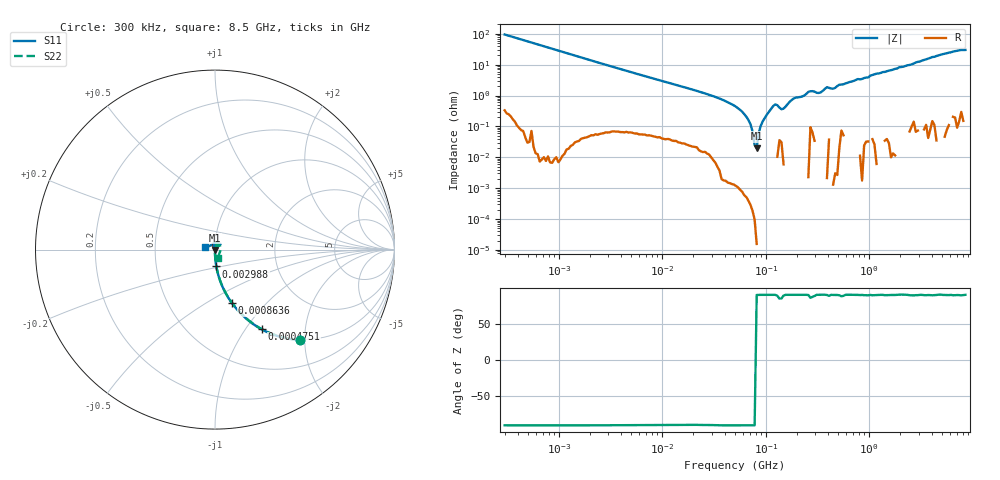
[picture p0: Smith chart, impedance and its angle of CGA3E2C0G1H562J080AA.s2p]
! S-parameter Generated by TDK Corporation
! Copyright(C) 2015 TDK Corporation.
! All Rights Reserved.
! TDK P/N: CGA3E2C0G1H562J080AA (Multilayer Ceramic Chip Capacitors)
! Property: C=5.6nF
! Size(LxWxT): 1.6x0.8x0.8mm, 0.063x0.031x0.031inches
! Model Type: s2p (Touchstone File Format Version 1.0)
! Frequency: DC=Yes Start=0.3MHz Stop=8500MHz 225points Log-sweep
! Note:
! Model Generated on Jun. 23, 2015
! Hash(MD5):
! Port Assignments:
!  1 ---| |--- 2
! Applicable Conditions:
!  Temperature = 25 degC
!  DC Bias Voltage = 0 V
!  Small Signal Operation
! Terms and conditions regarding TDK Simulation Models
! (1)This simulation model is being provided solely for informational purposes. Please refer to the specifications of the products in terms of detailed characteristics of such products.
! (2)In no event shall TDK Corporation of any of its subsidiaries be liable for any loss or damage arising, directly or indirectly,
!  From any information contained in this simulation model, including, but not limited to loss or damages arising from any inaccuracies, omissions or errors in connection with such information.
! (3)Any and all copyrights on this simulation model are owned by TDK Corporation.
!  Duplication or redistribution of this simulation model without prior written permission from TDK Corporation is prohibited.
! (4)This simulation model is subject to any modification or change without any prior notice.
! (5)Neither TDK Corporation nor any of its subsidiaries shall make any warranty, express or implied,
!  Including but not limited to the correctness, implied warranties of merchantability and fitness for a particular purpose with respect to this simulation models.
! (6)The use of this simulation model shall be deemed to have consented to the terms and conditions hereof.
# MHz S MA R 50
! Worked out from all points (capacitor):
!   224 points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, 300 kHz to 8.5 GHz, reference 50 ohm
!   read as one part in series: C = 5.6 nF near 314.1 kHz
!   lowest |Z| = 19.9 mohm at 81.83 MHz (marker M1)
!   series resonance near 80.2 MHz, so ESL is about 700 pH
!   S11 on the Smith chart (normalised r, x): 300 kHz: 0.99, -1.89; 475.1 kHz: 0.99, -1.19; 863.6 kHz: 0.99, -0.66; 2.988 MHz: 1.00, -0.19; 8.5 GHz: 0.90, +0.02
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0.3  0.6902 -46.8  0.7236 43.1  0.7236 43.5  0.6902 -46.7
0.47509  0.515 -59.6  0.8572 30.4  0.8572 30.5  0.515 -59.5
0.8636283  0.3131 -72.4  0.9495 17.8  0.9491 17.8  0.3132 -72.2
1.72111  0.1622 -81.6  0.9859 9.2  0.9824 9.2  0.1626 -81.3
2.988094  0.09404 -85.6  0.9951 5.4  0.9911 5.5  0.09444 -85.2
9.430415  0.0312 -89.2  0.9993 1.7  0.9967 1.9  0.0313 -89.9
51.67171  0.005867 -71.3  1 0.0  1 0.3  0.005867 -108.3
81.82903  0.002481 -46.8  1 -0.2  1 -0.0  0.002481 -133.4
102.9757  0.001212 -39.3  1 -0.4  1 -0.2  0.001212 -141.3
112.8926  0.0003362 -22.9  1 -0.6  1 -0.3  0.0003362 -158.0
178.7805  0.004567 42.9  1 -0.8  1 -0.5  0.004567 135.8
235.5662  0.00314 81.4  1 -1.1  1 -0.9  0.00314 96.6
283.1228  0.006416 81.4  0.9997 -1.4  0.9986 -1.0  0.006037 85.7
340.2802  0.001336 74.4  1 -1.6  1 -1.2  0.001336 102.8
390.6008  0.007426 92.6  0.9999 -2.0  0.9998 -1.5  0.00742 82.5
448.3627  0.001994 120.0  1 -1.8  1 -1.9  0.001994 56.3
514.6664  0.0064 80.2  0.9999 -2.2  0.9996 -2.2  0.006372 92.2
815.0429  0.004057 84.8  1 -3.7  0.9991 -3.4  0.004227 88.5
1551.304  0.007892 103.5  1 -6.7  1 -7.2  0.007892 62.6
2572.272  0.007551 104.7  1 -10.8  1 -12.0  0.007551 52.5
4073.536  0.04076 81.1  0.9986 -18.2  0.9975 -18.5  0.04051 59.5
8500  0.05545 167.2  0.9965 -38.9  0.9926 -38.6  0.0519 -71.2
